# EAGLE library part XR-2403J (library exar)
Enhanced MNP-5 modem MICROCONTROLLER
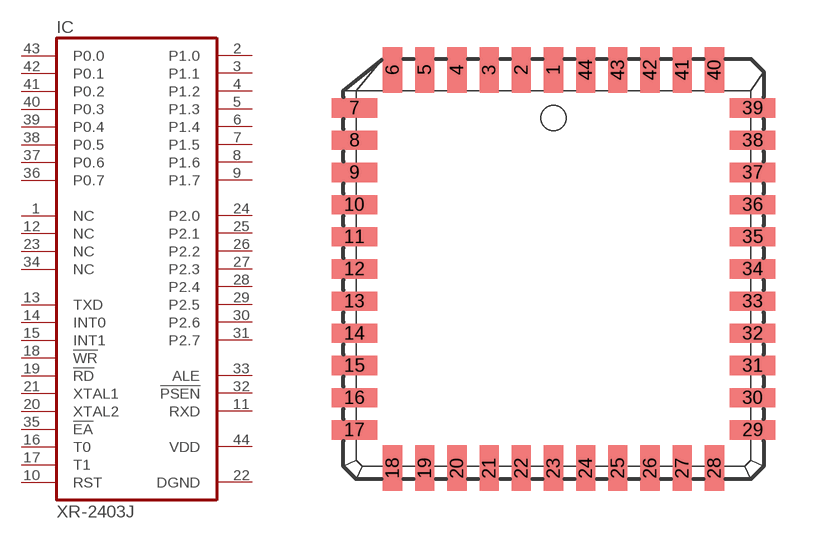
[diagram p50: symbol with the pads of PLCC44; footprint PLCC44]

Designator prefix IC

## XR-2403J (OC_FARNELL: unknown; OC_NEWARK: unknown)  [PLCC44]
1  NC  nc
2  P1.0
3  P1.1
4  P1.2
5  P1.3
6  P1.4
7  P1.5
8  P1.6
9  P1.7
10  RST  in
11  RXD  out
12  NC  nc
13  TXD  in
14  INT0  in
15  INT1  in
16  T0  in
17  T1  in
18  !WR  in
19  !RD  in
20  XTAL2  in
21  XTAL1  in
22  DGND  pwr
23  NC  nc
24  P2.0
25  P2.1
26  P2.2
27  P2.3
28  P2.4
29  P2.5
30  P2.6
31  P2.7
32  !PSEN  out
33  ALE  out
34  NC  nc
35  !EA  in
36  P0.7
37  P0.6
38  P0.5
39  P0.4
40  P0.3
41  P0.2
42  P0.1
43  P0.0
44  VDD  pwr

## Footprint PLCC44 (pad centres in mm)
Plastic Leaded Chip Carrier
smd 0.76 x 1.8: 1 0,7.86; 2 -1.27,7.86; 3 -2.54,7.86; 4 -3.81,7.86; 5 -5.08,7.86; 6 -6.35,7.86; 18 -6.35,-7.86; 19 -5.08,-7.86; 20 -3.81,-7.86; 21 -2.54,-7.86; 22 -1.27,-7.86; 23 0,-7.86; 24 1.27,-7.86; 25 2.54,-7.86; 26 3.81,-7.86; 27 5.08,-7.86; 28 6.35,-7.86; 40 6.35,7.86; 41 5.08,7.86; 42 3.81,7.86; 43 2.54,7.86; 44 1.27,7.86
smd 1.8 x 0.76: 7 -7.86,6.35; 8 -7.86,5.08; 9 -7.86,3.81; 10 -7.86,2.54; 11 -7.86,1.27; 12 -7.86,0; 13 -7.86,-1.27; 14 -7.86,-2.54; 15 -7.86,-3.81; 16 -7.86,-5.08; 17 -7.86,-6.35; 29 7.86,-6.35; 30 7.86,-5.08; 31 7.86,-3.81; 32 7.86,-2.54; 33 7.86,-1.27; 34 7.86,0; 35 7.86,1.27; 36 7.86,2.54; 37 7.86,3.81; 38 7.86,5.08; 39 7.86,6.35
